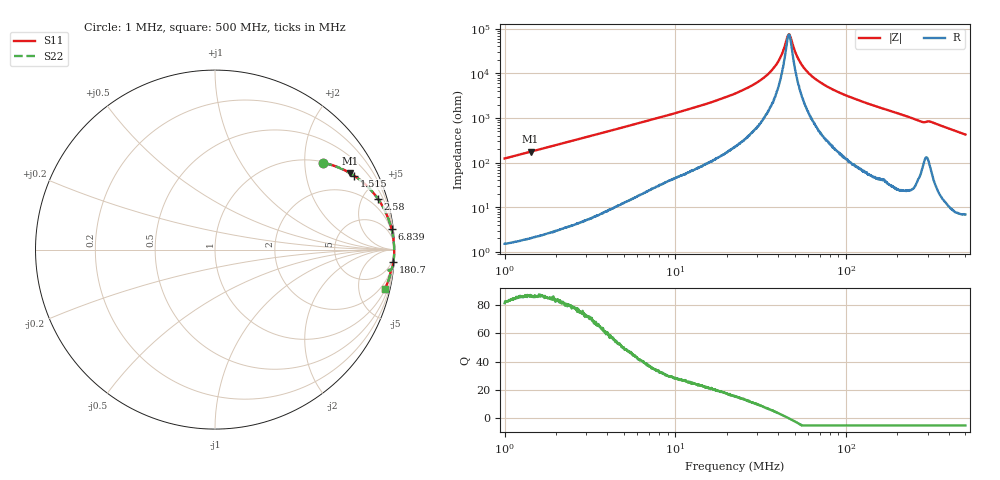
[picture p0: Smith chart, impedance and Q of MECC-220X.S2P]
!s-Parameter Generated by FASTRON Sdn. Bhd.
!FASTRON P/N : MECC-220X
!Keysight Technologies,E4991B,MY54100416,A.01.15
!Date: Wed Mar 18 10:26:37 2026
!Version  : Rev00 Wed Mar 18 10:26:37 2026
!Data & Calibration Information:
!PortZ  Port1:50+j0  Port2:50+j0
!When reading, reference impedance value at option line is always used.
!Remarks : This data is being provided solely for informational purposes.
!Freq	S11	S21	S12	S22
# Hz S dB R 50
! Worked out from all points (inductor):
!   1601 points, 1 MHz to 500 MHz, reference 50 ohm
!   read as one part in series: L = 19.7 uH near 1.032 MHz
!   highest Q = 86.7 at 1.418 MHz (marker M1), where L = 19.7 uH
!   self-resonance near 46.23 MHz
!   S11 on the Smith chart (normalised r, x): 1 MHz: 1.03, +2.48; 1.515 MHz: 1.04, +3.75; 2.58 MHz: 1.08, +6.39; 6.839 MHz: 1, +17; 180.7 MHz: 2, -29; 500 MHz: 1.14, -8.52
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1000000  -2.23 38.6  -4.09 -50.6  -4.09 -50.6  -2.23 38.6
1418460  -1.26 29.5  -6.16 -59.8  -6.16 -59.8  -1.26 29.5
1515283  -1.13 27.9  -6.59 -61.4  -6.59 -61.4  -1.13 27.9
2579841  -0.44 17.3  -10.53 -72.0  -10.53 -72.0  -0.44 17.3
2820919  -0.37 15.9  -11.25 -73.3  -11.25 -73.3  -0.37 15.9
6839020  -0.08 6.6  -18.78 -81.9  -18.78 -81.9  -0.08 6.6
7957584  -0.07 5.7  -20.13 -82.6  -20.13 -82.6  -0.07 5.7
2.236068e7  -0.02 1.6  -30.94 -84.7  -30.94 -84.7  -0.02 1.6
2.969105e7  -0.01 0.9  -35.65 -83.6  -35.65 -83.6  -0.01 0.9
3.605523e7  -0.01 0.5  -40.74 -79.9  -40.74 -79.9  -0.01 0.5
4.066875e7  -0.01 0.3  -46.29 -73.1  -46.29 -73.1  -0.01 0.3
4.516541e7  -0.01 0.1  -55.79 -33.8  -55.79 -33.8  -0.01 0.1
4.623034e7  -0.01 0.0  -57.13 -1.5  -57.13 -1.5  -0.01 0.0
4.750454e7  -0.01 -0.1  -55.80 34.7  -55.80 34.7  -0.01 -0.1
5.074715e7  -0.01 -0.2  -49.01 68.4  -49.01 68.4  -0.01 -0.2
5.358308e7  -0.01 -0.3  -45.22 75.9  -45.22 75.9  -0.01 -0.3
6.307767e7  -0.01 -0.7  -38.76 83.0  -38.76 83.0  -0.01 -0.7
9.229699e7  -0.01 -1.6  -31.25 85.9  -31.25 85.9  -0.01 -1.6
1.77937e8  -0.03 -3.9  -23.43 84.9  -23.43 84.9  -0.03 -3.9
1.807231e8  -0.03 -3.9  -23.26 84.8  -23.26 84.8  -0.03 -3.9
3.137236e8  -0.15 -6.8  -18.44 78.4  -18.44 78.4  -0.15 -6.8
5e8  -0.26 -13.2  -12.85 75.9  -12.85 75.9  -0.26 -13.2
